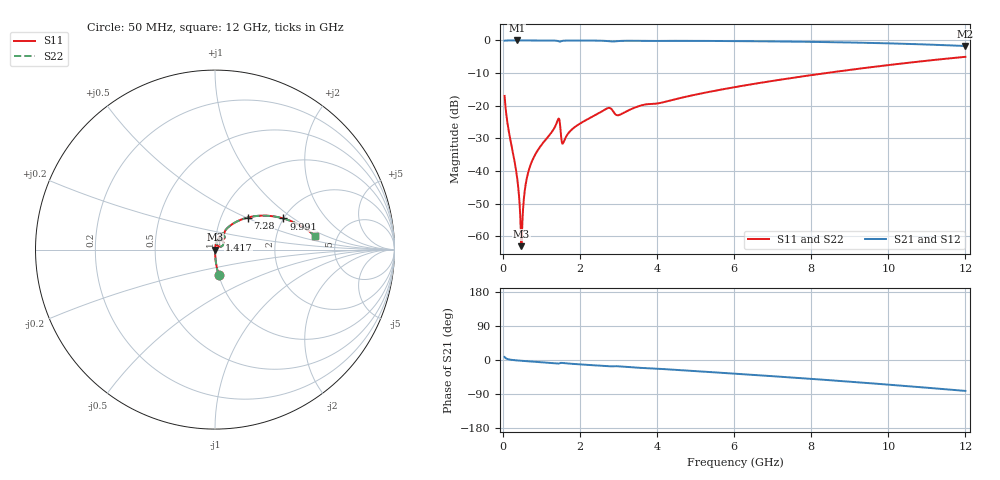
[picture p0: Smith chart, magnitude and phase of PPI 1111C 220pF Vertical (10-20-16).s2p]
# GHz S MA R 50
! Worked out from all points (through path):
!   1601 points, 50 MHz to 12 GHz, reference 50 ohm
!   highest |S21| = -0.01 dB at 363.7 MHz (marker M1); lowest = -1.7 dB at 12 GHz (marker M2)
!   group delay of S21, straight-line fit = 18.8 ps
!   lowest |S11| = -63.0 dB at 483.2 MHz (marker M3), VSWR 1.00, Z = 50.1 - j0.0194 ohm
!   |S11| at or under -10 dB: start of sweep to 8.38 GHz
!   |S22| runs from -63.0 to -5.0 dB; largest |S21 - S12| = 0
!   S11 on the Smith chart (normalised r, x): 50 MHz: 1.00, -0.29; 1.417 GHz: 1.04, +0.11; 7.28 GHz: 1.33, +0.51; 9.991 GHz: 2.00, +0.84; 12 GHz: 3.38, +0.76
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0.05  0.1414 -82.0  0.9897 7.9  0.9897 7.9  0.1414 -82.0
0.3636875  0.008798 -87.1  0.9993 -1.0  0.9993 -1.0  0.008798 -87.1
0.4458437  0.002667 -77.3  0.9993 -1.7  0.9993 -1.7  0.002667 -77.3
0.4831875  0.0007097 -15.9  0.9993 -2.0  0.9993 -2.0  0.0007097 -15.9
0.528  0.002601 71.6  0.9992 -2.4  0.9992 -2.4  0.002601 71.6
0.5728125  0.005037 78.8  0.9992 -2.7  0.9992 -2.7  0.005037 78.8
0.617625  0.007361 80.9  0.9992 -3.0  0.9992 -3.0  0.007361 80.9
0.737125  0.01311 82.4  0.999 -3.9  0.999 -3.9  0.01311 82.4
1.416781  0.05785 66.7  0.9843 -9.2  0.9843 -9.2  0.05785 66.7
1.454125  0.06376 51.1  0.9669 -9.3  0.9669 -9.3  0.06376 51.1
1.581094  0.02789 62.8  0.9905 -8.2  0.9905 -8.2  0.02789 62.8
1.767813  0.0419 76.2  0.9961 -9.9  0.9961 -9.9  0.0419 76.2
2.044156  0.05513 75.8  0.9961 -11.8  0.9961 -11.8  0.05513 75.8
2.723813  0.09204 62.0  0.9776 -16.7  0.9776 -16.7  0.09204 62.0
3.000156  0.07166 58.9  0.9794 -16.6  0.9794 -16.6  0.07166 58.9
4.038312  0.1091 60.9  0.9825 -23.2  0.9825 -23.2  0.1091 60.9
6.025  0.1931 52.8  0.9771 -36.1  0.9771 -36.1  0.1931 52.8
7.27975  0.2548 44.5  0.9628 -44.7  0.9628 -44.7  0.2548 44.5
8.019156  0.2953 39.3  0.951 -49.9  0.951 -49.9  0.2953 39.3
9.990906  0.4188 24.5  0.903 -64.9  0.903 -64.9  0.4188 24.5
10.01331  0.4203 24.3  0.9023 -65.1  0.9023 -65.1  0.4203 24.3
12  0.5618 7.9  0.8212 -81.6  0.8212 -81.6  0.5618 7.9
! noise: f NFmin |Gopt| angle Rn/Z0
0.05  0.0003684  0.8648  0.2985  0.0005851
1.372  0.009045  0.8503  5.768  0.01284
2.701  0.01985  0.8654  11.33  0.03135
4.031  0.02088  0.8159  16.76  0.02321
5.36  0.01417  0.6721  21.53  0.008042
6.682  0.01537  0.6371  26.19  0.007592
8.012  0.01742  0.6265  30.74  0.008153
9.341  0.01988  0.6274  35.15  0.009134
10.67  0.02273  0.6361  39.43  0.01049
12  0.02605  0.6509  43.62  0.01231
